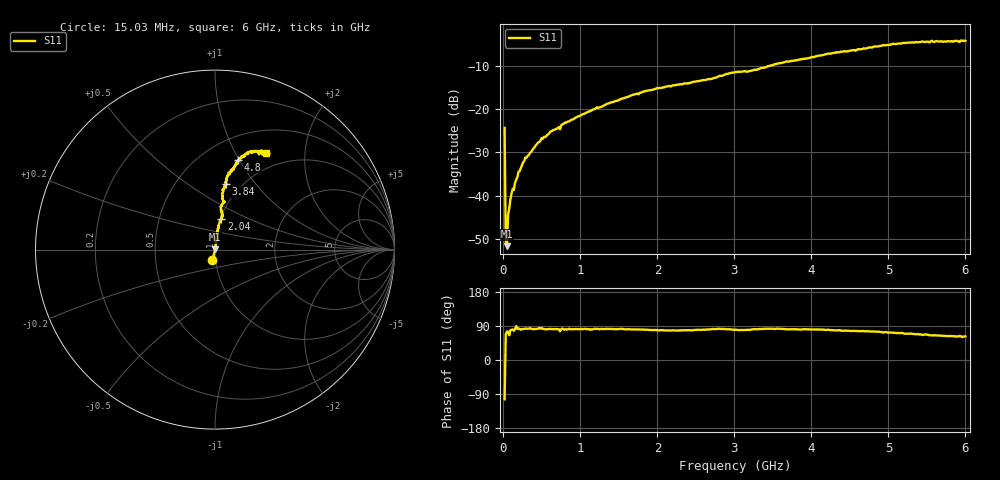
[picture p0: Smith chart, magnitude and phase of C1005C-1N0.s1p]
!	Network	Analyzer	HP8753E.07.74:	Oct	30	2002	Serial	No.	JP38451487
!	Hewlett-Packard
!	7	Sep	2009	8:16:31
!	Frequency	S11
#	HZ	S	RI	R	50
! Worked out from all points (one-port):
!   400 points, 15.03 MHz to 6 GHz, reference 50 ohm
!   lowest |S11| = -51.6 dB at 45.03 MHz (marker M1), VSWR 1.01, Z = 50.1 + j0.255 ohm
!   |S11| at or under -10 dB: start of sweep to 3.463 GHz
!   S11 on the Smith chart (normalised r, x): 15.03 MHz: 0.96, -0.11; 2.04 GHz: 1.01, +0.36; 3.84 GHz: 0.85, +0.72; 4.8 GHz: 0.73, +0.99; 6 GHz: 0.78, +1.34
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1.502992e7  -0.0145 -0.0589
3.002985e7  0.00114 0.00279
4.502978e7  0.000674 0.00255
6.00297e7  0.00161 0.00578
9.002955e7  0.00178 0.00889
1.200294e8  0.00201 0.0119
1.350293e8  0.00261 0.0114
1.500292e8  0.00199 0.014
1.95029e8  0.00214 0.0188
2.850286e8  0.0033 0.0275
4.950275e8  0.0041 0.0462
7.200264e8  0.00937 0.0615
7.350263e8  0.0144 0.0567
7.650262e8  0.00788 0.0663
1.215024e9  0.0143 0.104
1.515022e9  0.0175 0.127
2.04002e9  0.0353 0.171
2.265019e9  0.0394 0.187
3.015015e9  0.0474 0.263
3.765011e9  0.0536 0.355
3.840011e9  0.0624 0.366
4.515007e9  0.111 0.46
4.800006e9  0.129 0.501
5.265004e9  0.205 0.546
5.865001e9  0.285 0.542
5.925e9  0.262 0.53
5.955e9  0.304 0.534
6e9  0.285 0.539
